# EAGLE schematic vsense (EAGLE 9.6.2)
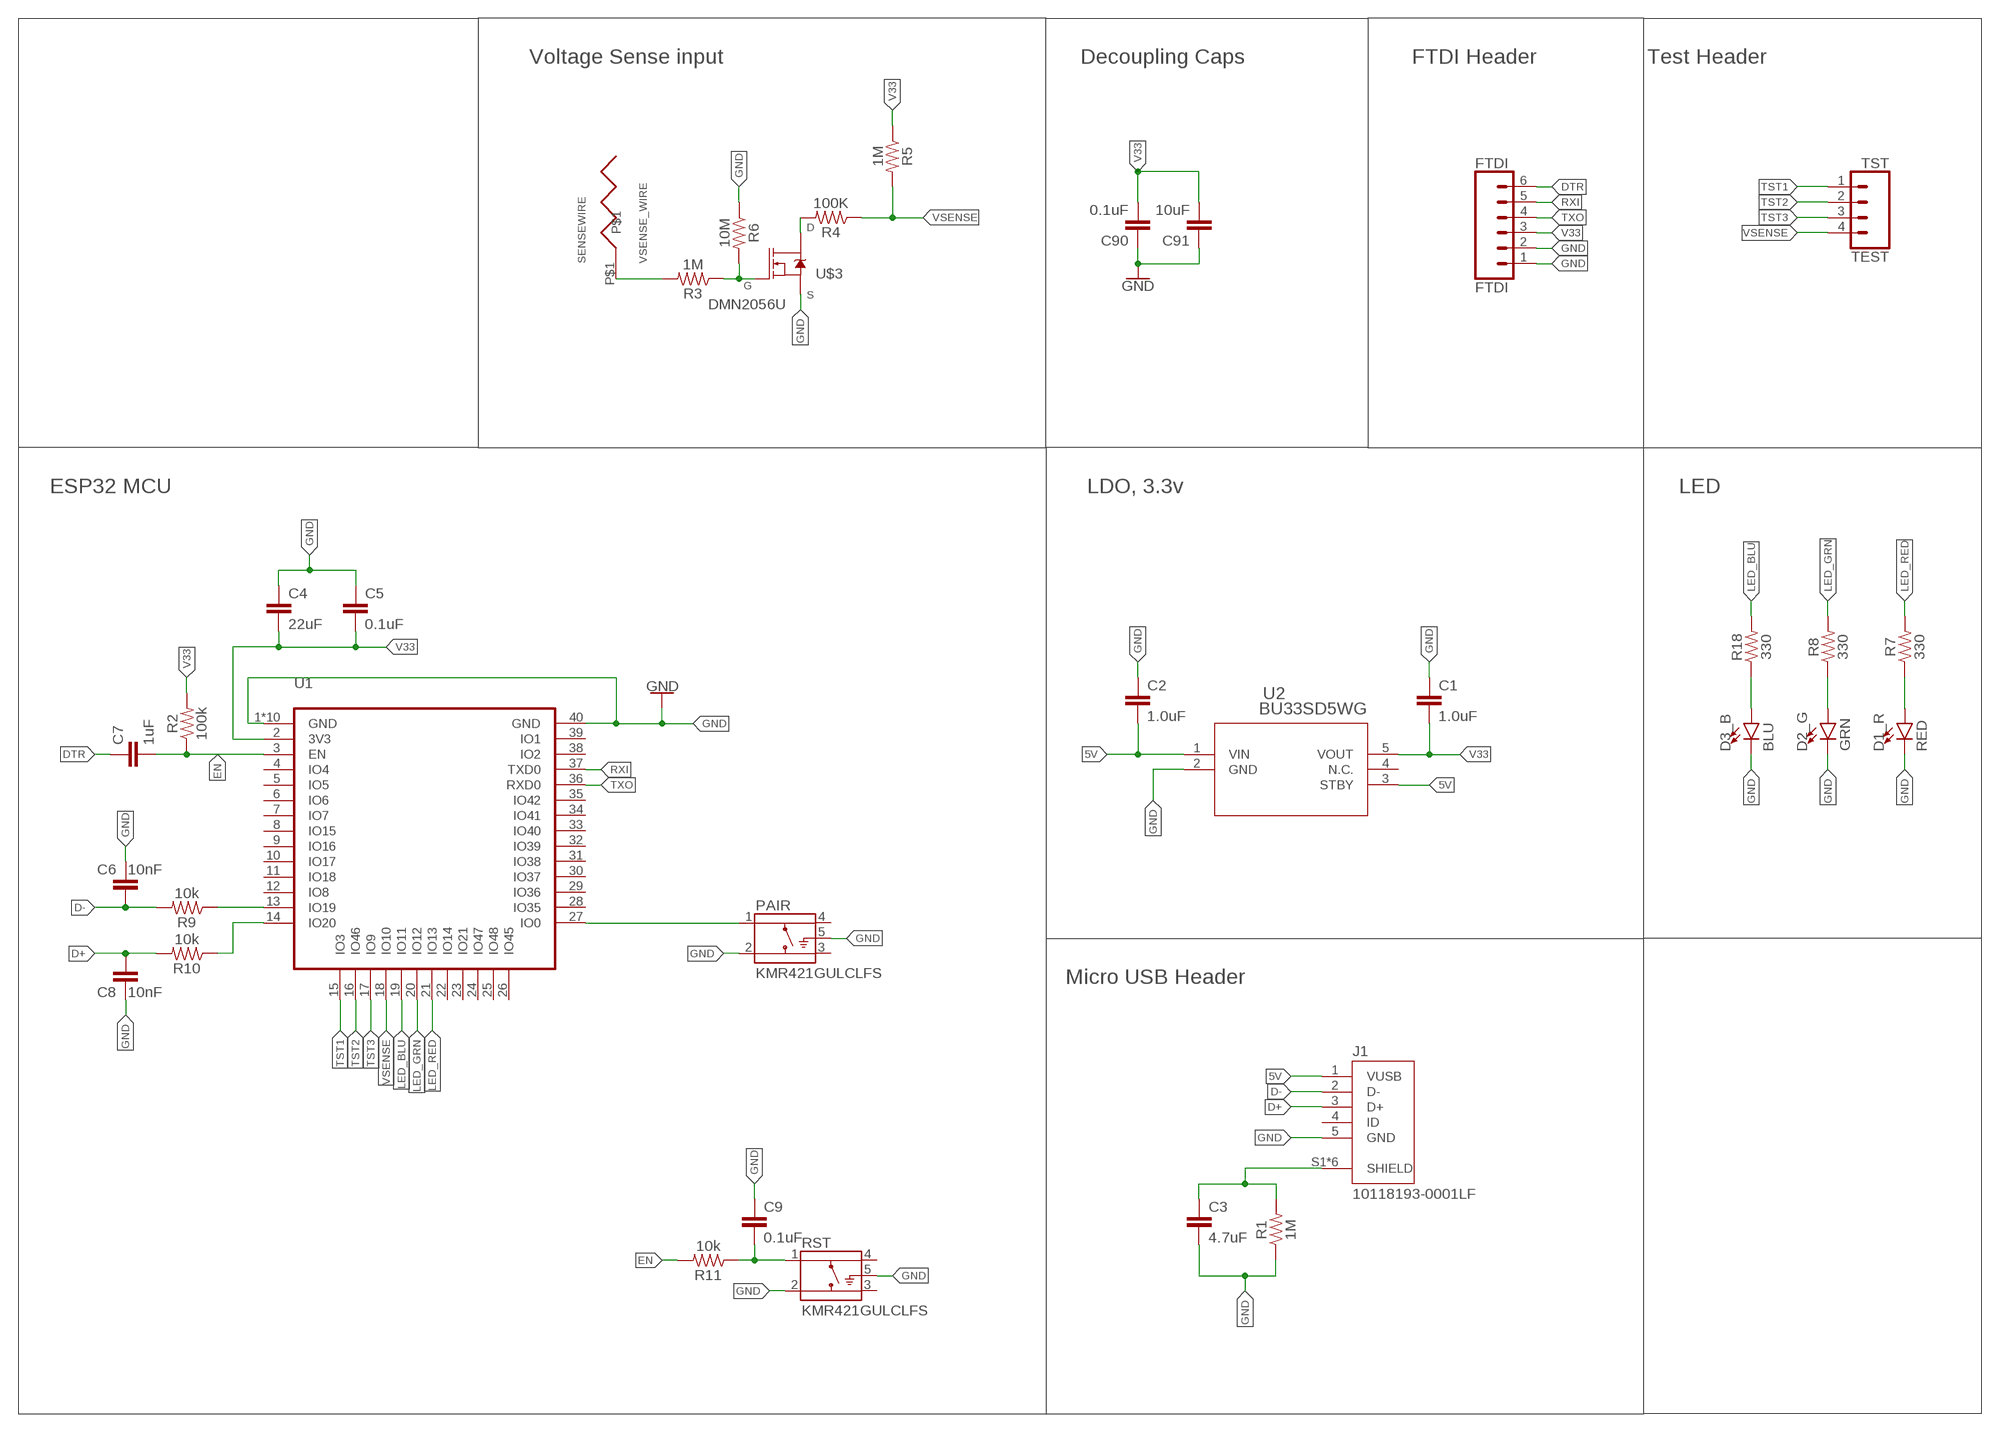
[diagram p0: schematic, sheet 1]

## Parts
C1  1.0uF  1.0UF-0603-16V-10%  [0603]
C2  1.0uF  1.0UF-0603-16V-10%  [0603]
C3  4.7uF  4.7UF0603  [0603]
C4  22uF  1.0UF-0603-16V-10%  [0603]
C5  0.1uF  1.0UF-0603-16V-10%  [0603]
C6  10nF  1.0UF-0603-16V-10%  [0603]
C7  1uF  1.0UF-0603-16V-10%  [0603]
C8  10nF  1.0UF-0603-16V-10%  [0603]
C9  0.1uF  1.0UF-0603-16V-10%  [0603]
C90  0.1uF  0.1UF-0603-25V-5%  [0603]
C91  10uF  10UF-0603-6.3V-20%  [0603]
D1_R  RED  LED-SMD0603  [LED-0603]
D2_G  GRN  LED-SMD0603  [LED-0603]
D3_B  BLU  LED-SMD0603  [LED-0603]
FTDI  FTDI  CONN_06SILK_FEMALE_PTH  [1X06]
J1  10118193-0001LF  [FCI_10118193-0001LF]
PAIR  KMR421GULCLFS  [SW_KMR421GULCLFS]
R1  1M  RESISTOR0603  [0603]
R2  100k  RESISTOR0603  [0603]
R3  1M  RESISTOR0603  [0603]
R4  100K  RESISTOR0603  [0603]
R5  1M  RESISTOR0603  [0603]
R6  10M  RESISTOR0603  [0603]
R7  330  330OHM-0603-1/10W-1%  [0603]
R8  330  330OHM-0603-1/10W-1%  [0603]
R9  10k  RESISTOR0603  [0603]
R10  10k  RESISTOR0603  [0603]
R11  10k  RESISTOR0603  [0603]
R18  330  330OHM-0603-1/10W-1%  [0603]
RST  KMR421GULCLFS  [SW_KMR421GULCLFS]
SENSEWIRE  VSENSE_WIRE  [VSENSE_WIRE]
TEST  TST  CONN_04  [1X04]
U1  ESP32-S3-WROOM-1  [ESP32-S3-WROOM-1]
U2  BU33SD5WG  BU33SD5WG-TR  [SSOP5_ROM]
U$3  DMN2056U  [SOT23-3]

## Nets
5V: C2.2 J1.1(VUSB) U2.1(VIN) U2.3(STBY)
D+: C8.2 J1.3(D+) R10.2
D-: C6.1 J1.2(D-) R9.2
DTR: C7.1 FTDI.6
EN: C7.2 R2.1 R11.2 U1.3(EN)
GND: C1.1 C2.1 C3.2 C4.1 C5.1 C6.2 C8.1 C9.1 C90.1 C91.1 D1_R.C D2_G.C D3_B.C FTDI.1 FTDI.2 J1.5(GND) PAIR.2 PAIR.5(G) R1.1 R6.1 RST.2 RST.5(G) U1.1(GND) U1.40(GND) U1.P$1(GND) U1.P$2(GND) U1.P$3(GND) U1.P$4(GND) U1.P$5(GND) U1.P$6(GND) U1.P$7(GND) U1.P$8(GND) U1.P$9(GND) U2.2(GND) U$3.2(S)
LED_BLU: R18.2 U1.19(IO11)
LED_GRN: R8.2 U1.20(IO12)
LED_RED: R7.2 U1.21(IO13)
N$1: R4.2 U$3.3(D)
N$2: PAIR.1 U1.27(IO0)
N$3: C3.1 J1.S1(SHIELD) J1.S2(SHIELD) J1.S3(SHIELD) J1.S4(SHIELD) J1.S5(SHIELD) J1.S6(SHIELD) R1.2
N$4: R3.1 R6.2 U$3.1(G)
N$5: C9.2 R11.1 RST.1
N$6: D2_G.A R8.1
N$7: R3.2 SENSEWIRE.P$1
N$8: D3_B.A R18.1
N$9: R9.1 U1.13(IO19)
N$10: R10.1 U1.14(IO20)
N$19: D1_R.A R7.1
RXI: FTDI.5 U1.37(TXD0)
TST1: TEST.1 U1.15(IO3)
TST2: TEST.2 U1.16(IO46)
TST3: TEST.3 U1.17(IO9)
TXO: FTDI.4 U1.36(RXD0)
V33: C1.2 C4.2 C5.2 C90.2 C91.2 FTDI.3 R2.2 R5.1 U1.2(3V3) U2.5(VOUT)
VSENSE: R4.1 R5.2 TEST.4 U1.18(IO10)
Unconnected: J1.4(ID) PAIR.3 PAIR.4 RST.3 RST.4 U1.4(IO4) U1.5(IO5) U1.6(IO6) U1.7(IO7) U1.8(IO15) U1.9(IO16) U1.10(IO17) U1.11(IO18) U1.12(IO8) U1.22(IO14) U1.23(IO21) U1.24(IO47) U1.25(IO48) U1.26(IO45) U1.28(IO35) U1.29(IO36) U1.30(IO37) U1.31(IO38) U1.32(IO39) U1.33(IO40) U1.34(IO41) U1.35(IO42) U1.38(IO2) U1.39(IO1) U2.4(N.C.)

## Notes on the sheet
- Voltage Sense input | Decoupling Caps | FTDI Header | Test Header
- ESP32 MCU | LDO, 3.3v | LED
- Micro USB Header

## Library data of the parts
C1 C2 = SparkFun-Capacitors:1.0UF: 1µF ceramic capacitors; PROD_ID: CAP-00868
C3 = SparkFun-Capacitors:4.7UF: 4.7µF ceramic capacitors; PROD_ID: CAP-08280
C4-C9 = SparkFun-Capacitors:1.0UF: 1µF ceramic capacitors; PROD_ID: CAP-00868; VALUE: 1.0uF
C90 = SparkFun-Capacitors:0.1UF: 0.1µF ceramic capacitors; PROD_ID: CAP-08604
C91 = SparkFun-Capacitors:10UF: 10.0µF ceramic capacitors; PROD_ID: CAP-11015
D1_R = siguino:LED-SMD: Red SMD LED; PROD_ID: DIO-00819
D2_G D3_B = siguino:LED-SMD: Red SMD LED; PROD_ID: DIO-00819; VALUE: RED
FTDI = SparkFun-Connectors:CONN_06: Multi connection point. Often used as Generic Header-pin footprint for 0.1 inch spaced/style header connections On any of the 0.1 inch spaced packages, you can populate with these: Break Away Headers - Straight (PRT-00116) Break Away Male Headers - Right Angle (PRT-00553) Female Headers (PRT-00115)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; PROD_ID: CONN-08437
J1 = siguino:10118193-0001LF: Micro USB B Type Receptacle; DESCRIPTION: Single Port 5 Contact Shielded SMT MICRO USB B-Type Receptacle; DIGI-KEY_PART_NUMBER: 609-4616-1-ND; DIGI-KEY_PURCHASE_URL: https://www.digikey.ie/product-detail/en/amphenol-fci/10118193-0001LF/609-4616-1-ND/2785380?utm_source=snapeda&utm_medium=aggregator&utm_campaign=symbol; MF: Amphenol FCI; MP: 10118193-0001LF; PACKAGE: None
PAIR RST = siguino:KMR421GULCLFS: Switch Tactile N.O. SPST Round Button Gull Wing 0.05A 32VDC 1VA 200000Cycles 2N SMD Automotive T/R; DESCRIPTION: Tactile Switch SPST-NO Top Actuated Surface Mount; DIGI-KEY_PART_NUMBER: CKN12152CT-ND; DIGIKEY-PURCHASE-URL: https://snapeda.com/shop?store=DigiKey&id=668006; MF: C&K; MP: KMR421GULCLFS; PACKAGE: None
R1-R6 R9-R11 = SparkFun-Resistors:RESISTOR: Generic Resistor Package
R7 R8 R18 = SparkFun-Resistors:330OHM: 330Ω resistor; PROD_ID: RES-00818
SENSEWIRE = siguino:VSENSE_WIRE: External wire with single input for voltage sensing
TEST = SparkFun-Connectors:CONN_04: Multi connection point. Often used as Generic Header-pin footprint for 0.1 inch spaced/style header connections On any of the 0.1 inch spaced packages, you can populate with these: Break Away Headers - Straight (PRT-00116) Break Away Male Headers - Right Angle (PRT-00553) Female Headers (PRT-00115)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; PROD_ID: CONN-09696
U1 = ESP32-S3-WROOM-1:ESP32-S3-WROOM-1: ESP32-S3-WROOM-1 WiFi Module Check availability; AVAILABILITY: In Stock; DESCRIPTION: SMD MODULE, ESP32-S3R8 WITH 8 MB; MF: Espressif Systems; MP: ESP32-S3-WROOM-1; PACKAGE: None; PRICE: None; PURCHASE-URL: https://pricing.snapeda.com/search/part/ESP32-S3-WROOM-1/?ref=eda
U2 = siguino:BU33SD5WG-TR; BUILT_BY: EMA_Molly; COPYRIGHT: Copyright (C) 2018 Accelerated Designs. All rights reserved; MANUFACTURER_PART_NUMBER: BU33SD5WG-TR; SOURCELIBRARY: ROHM_2019-10-21; VENDOR: ROHM Semiconductor
U$3 = siguino:DMN2056U: Diodes Incorporated NCH MOSFET This MOSFET is designed to minimize the on-state resistance (RDS(ON)) and yet maintain superior switching performance, making it ideal for high efficiency power management applications.

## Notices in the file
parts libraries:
SparkFun-Capacitors: Licensing: Creative Commons ShareAlike 4.0 International - https://creativecommons.org/licenses/by-sa/4.0
